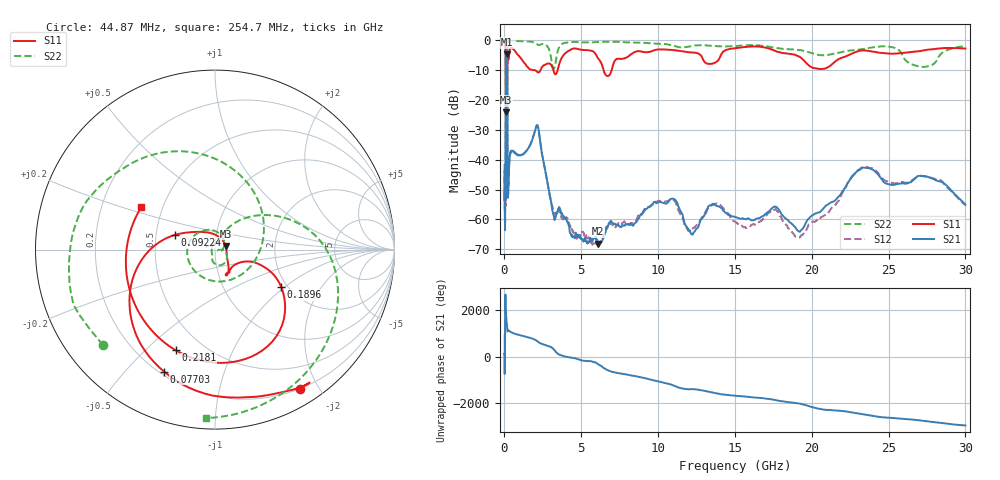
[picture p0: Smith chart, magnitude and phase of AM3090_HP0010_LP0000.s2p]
! Date/Time: Thu, Feb 28, 2019 1:54 PM
! Network Analyzer: Agilent Technologies E8364B Rev: A.07.50.67
! Sweep from 0.010 to 30.000 GHz, 1601 Points, Sweep Type: LOG
! Power Supply: 5.023 V, 0.002 A
# Hz S DB R 50
!freq MagS11 AngS11 MagS21 AngS21 MagS12 AngS12 MagS22 AngS22
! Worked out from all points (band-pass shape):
!   1601 points, 10 MHz to 30 GHz, reference 50 ohm
!   highest |S21| = -4.79 dB at 134.9 MHz (marker M1); lowest = -68.1 dB at 6.11 GHz (marker M2)
!   |S21| within 3 dB of the highest: 99.81 MHz to 174.3 MHz (74.47 MHz wide, 54.3 % of centre)
!   lowest |S11| = -24.1 dB at 99.43 MHz (marker M3), VSWR 1.13, Z = 56.2 + j2.26 ohm
!   |S11| at or under -10 dB: 1.811 GHz to 2.352 GHz (540.5 MHz wide, 26 % of centre); 3.18 GHz to 3.465 GHz (285.2 MHz wide, 8.58 % of centre); 6.451 GHz to 6.979 GHz (528.2 MHz wide, 7.87 % of centre)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
!   |S22| runs from -35.7 to -0.1 dB; largest |S21 - S12| = 0.012
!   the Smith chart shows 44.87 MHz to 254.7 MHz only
!   S11 on the Smith chart (normalised r, x): 44.87 MHz: 0.20, -1.76; 77.03 MHz: 0.22, -0.64; 92.24 MHz: 0.63, +0.11; 189.6 MHz: 1.86, -0.94; 218.1 MHz: 0.35, -0.62; 254.7 MHz: 0.38, +0.23
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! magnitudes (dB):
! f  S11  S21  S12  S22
! 10 MHz  -0.2  -41.8  -45.6  -0.5
! 38.04 MHz  -0.5  -62.6  -62.3  -1.3
! 44.87 MHz  -0.8  -54.7  -54.1  -1.7
! 69.7 MHz  -1.9  -51.8  -54.4  -3.4
! 77.03 MHz  -2.7  -45.3  -44.3  -5.2
! 92.24 MHz  -12.4  -13.9  -13.9  -15.3
! 99.43 MHz  -24.1  -7.9  -7.9  -16.9
! 134.9 MHz  -16.6  -4.8  -4.8  -30.4
! 144.7 MHz  -16.4  -4.9  -4.9  -21.6
! 169.8 MHz  -15.4  -6.8  -6.8  -34.9
! 189.6 MHz  -7.5  -19.1  -19.1  -10.0
! 218.1 MHz  -4.4  -52.6  -51.5  -1.5
! 254.7 MHz  -6.5  -50.5  -49.1  -0.5
! 550.5 MHz  -3.0  -37.0  -37.3  -0.2
! 2.084 GHz  -10.5  -28.8  -28.7  -1.3
! 3.22 GHz  -10.7  -59.1  -57.8  -9.6
! 6.11 GHz  -6.2  -68.1  -67.4  -0.6
! 7.926 GHz  -5.9  -61.5  -61.2  -0.8
! 10.65 GHz  -3.3  -54.2  -53.9  -1.5
! 19.22 GHz  -5.6  -64.1  -66.0  -3.3
! 23.48 GHz  -3.5  -42.7  -42.4  -2.9
! 30 GHz  -2.8  -55.1  -55.1  -2.2
